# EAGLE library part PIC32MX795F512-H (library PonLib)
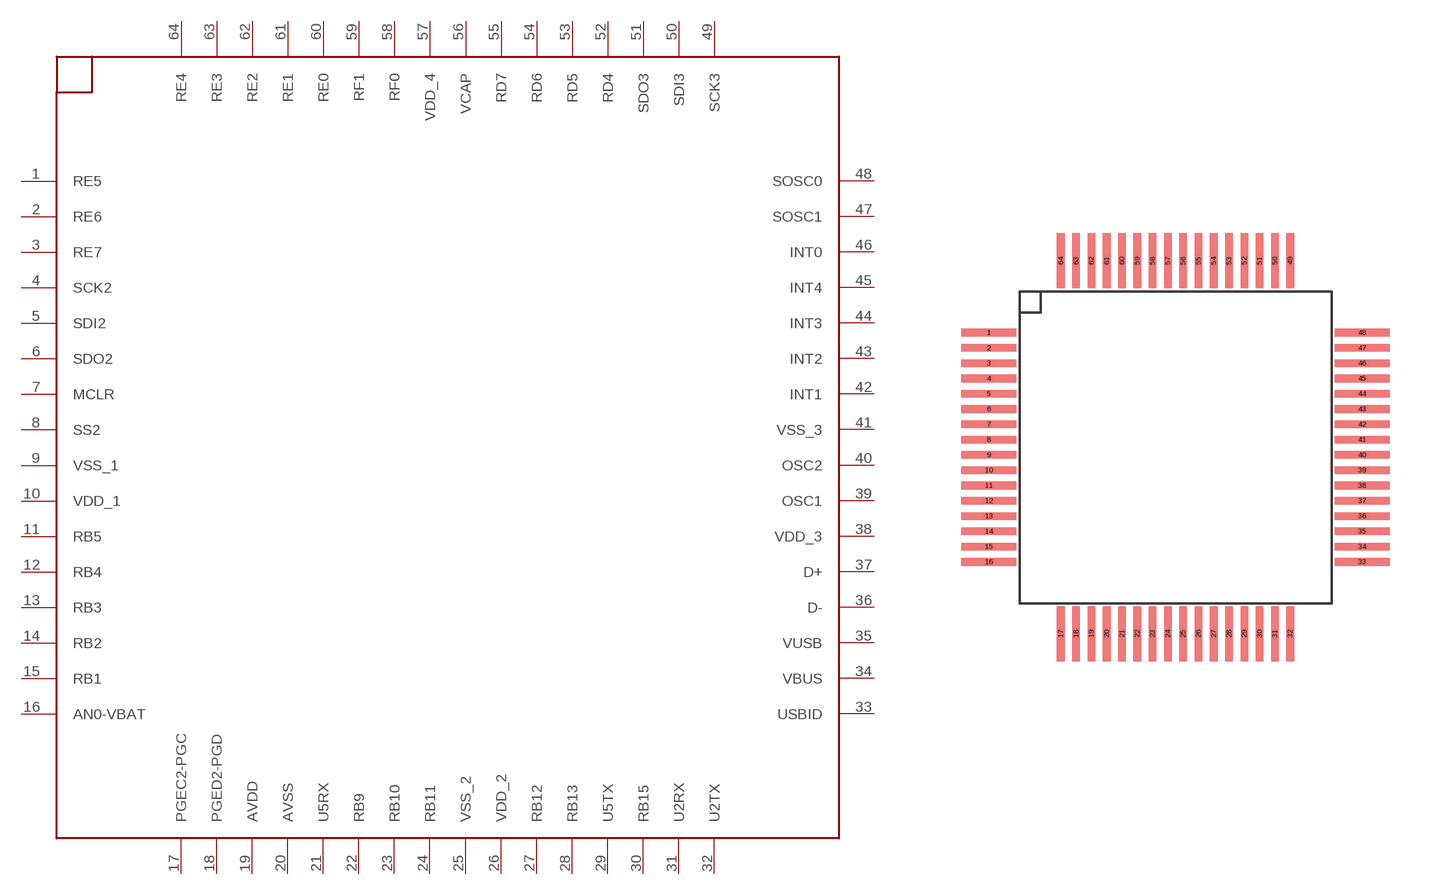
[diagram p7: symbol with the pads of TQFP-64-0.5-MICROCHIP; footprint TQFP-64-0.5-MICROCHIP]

Designator prefix -

## PIC32MX795F512-H  [TQFP-64-0.5-MICROCHIP]
1  RE5
2  RE6
3  RE7
4  SCK2
5  SDI2
6  SDO2
7  MCLR
8  SS2
9  VSS_1
10  VDD_1
11  RB5
12  RB4
13  RB3
14  RB2
15  RB1
16  AN0-VBAT
17  PGEC2-PGC
18  PGED2-PGD
19  AVDD
20  AVSS
21  U5RX
22  RB9
23  RB10
24  RB11
25  VSS_2
26  VDD_2
27  RB12
28  RB13
29  U5TX
30  RB15
31  U2RX
32  U2TX
33  USBID
34  VBUS
35  VUSB
36  D-
37  D+
38  VDD_3
39  OSC1
40  OSC2
41  VSS_3
42  INT1
43  INT2
44  INT3
45  INT4
46  INT0
47  SOSC1
48  SOSC0
49  SCK3
50  SDI3
51  SDO3
52  RD4
53  RD5
54  RD6
55  RD7
56  VCAP
57  VDD_4
58  RF0
59  RF1
60  RE0
61  RE1
62  RE2
63  RE3
64  RE4

## Footprint TQFP-64-0.5-MICROCHIP (pad centres in mm)
smd 1.8 x 0.25: 1 -6.1,3.75; 2 -6.1,3.25; 3 -6.1,2.75; 4 -6.1,2.25; 5 -6.1,1.75; 6 -6.1,1.25; 7 -6.1,0.75; 8 -6.1,0.25; 9 -6.1,-0.25; 10 -6.1,-0.75; 11 -6.1,-1.25; 12 -6.1,-1.75; 13 -6.1,-2.25; 14 -6.1,-2.75; 15 -6.1,-3.25; 16 -6.1,-3.75; 33 6.1,-3.75; 34 6.1,-3.25; 35 6.1,-2.75; 36 6.1,-2.25; 37 6.1,-1.75; 38 6.1,-1.25; 39 6.1,-0.75; 40 6.1,-0.25; 41 6.1,0.25; 42 6.1,0.75; 43 6.1,1.25; 44 6.1,1.75; 45 6.1,2.25; 46 6.1,2.75; 47 6.1,3.25; 48 6.1,3.75
smd 0.25 x 1.8: 17 -3.75,-6.1; 18 -3.25,-6.1; 19 -2.75,-6.1; 20 -2.25,-6.1; 21 -1.75,-6.1; 22 -1.25,-6.1; 23 -0.75,-6.1; 24 -0.25,-6.1; 25 0.25,-6.1; 26 0.75,-6.1; 27 1.25,-6.1; 28 1.75,-6.1; 29 2.25,-6.1; 30 2.75,-6.1; 31 3.25,-6.1; 32 3.75,-6.1; 49 3.75,6.1; 50 3.25,6.1; 51 2.75,6.1; 52 2.25,6.1; 53 1.75,6.1; 54 1.25,6.1; 55 0.75,6.1; 56 0.25,6.1; 57 -0.25,6.1; 58 -0.75,6.1; 59 -1.25,6.1; 60 -1.75,6.1; 61 -2.25,6.1; 62 -2.75,6.1; 63 -3.25,6.1; 64 -3.75,6.1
